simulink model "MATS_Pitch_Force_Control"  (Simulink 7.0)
settings: Solver=FixedStepDiscrete  StartTime=0.0  StopTime=inf  RelTol=1e-3
PreLoadFcn:
  | scramInitialize
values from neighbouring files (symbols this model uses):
  node = completenodestruct(node)    [scramInitialize.m]
  nTbl = 6    [scramInitialize.m]
  samplePeriod = 1/1024    (= 0.0009765625)    [scramInitialize.m]    (also in viewer.m = eval(getHeaderValue(header, 'DELTA_T')))
undefined symbols (not defined in the file or in its folder): DiscIntNeverNeededParam
libraries: xpcsystranlib x3, xpclib x2

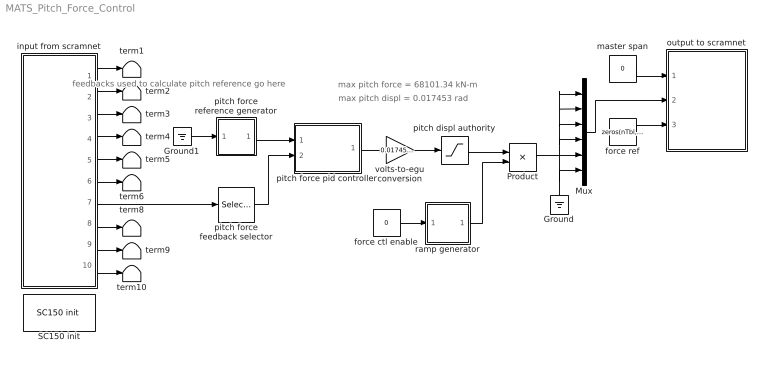
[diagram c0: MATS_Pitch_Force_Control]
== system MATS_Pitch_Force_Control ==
  note: max pitch displ = 0.017453 rad
  note: max pitch force = 68101.34 kN-m
  note: feedbacks used to calculate pitch reference go here
  Ground : Ground  Orientation=up
  Ground1 : Ground
  Mux : Mux  Inputs=nTbl
  Product : Product  OutDataType=sfix(16)  OutScaling=2^0
  SC150 init : xpcsystranlib/Shared Memory/SC150 init   node=node  pci=-1
  force ctl enable : Constant  Value=0  OutDataType=sfix(16)  OutScaling=2^0
  force ref : Constant  Value=zeros(nTbl, 1)  OutDataType=sfix(16)  OutScaling=2^0
  input from scramnet : Subsystem
  master span : Constant  Value=0  OutDataType=sfix(16)  OutScaling=2^0
  output to scramnet : Subsystem
  pitch displ authority : Saturate  UpperLimit=0.017453  LowerLimit=-0.017453  OutDataType=sfix(16)  OutScaling=2^0
  pitch force feedback selector : Selector  IndexOptions=Index vector (dialog)  Indices=5  OutputSizes=1
  pitch force pid controller : Subsystem  mask(Proportional-Integral-Derivative (PID) Controller){kp=0.1, ki=0, maxAuthority=5, kd=0, kf=0, bw=1/samplePeriod, maxUnits=68101.34, samplePeriod=samplePeriod}
      mask prompts: kp "Proportional gain"; ki "Integral gain"; maxAuthority "Max authority (percent)"; kd "Derivative gain"; kf "Feedforward gain"; bw "Bandwidth (Hz)"; maxUnits "Max units"; samplePeriod "Sample period (sec)"
  pitch force reference generator : Subsystem
  ramp generator : Subsystem  mask{rate=100}
      mask prompts: rate "Ramp rate (%/sec)"
  term{1..6,8..10} (9 alike) : Terminator
  volts-to-egu conversion : Gain  Gain=0.017453 / 10  ParameterDataType=sfix(16)  ParameterScaling=2^0  OutDataType=sfix(16)  OutScaling=2^0
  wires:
  master span/1 -> output to scramnet/1(master span)
  input from scramnet/1(master span) -> term1/1
  input from scramnet/2(displ ref) -> term2/1
  input from scramnet/3(veloc ref) -> term3/1
  input from scramnet/5(displ fbk) -> term5/1
  input from scramnet/6(veloc fbk) -> term6/1
  input from scramnet/7(force fbk) -> pitch force feedback selector/1
  input from scramnet/8(comp fbk) -> term8/1
  input from scramnet/9(press fbk) -> term9/1
  input from scramnet/10(user adcs) -> term10/1
  Ground/1 -> Mux/6, Mux/1, Mux/2, Mux/3, Mux/4
  pitch force feedback selector/1 -> pitch force pid controller/2(fbk)
  pitch force reference generator/1(out) -> pitch force pid controller/1(cmd)
  force ctl enable/1 -> ramp generator/1(inp)
  ramp generator/1(out) -> Product/2
  pitch force pid controller/1(out) -> volts-to-egu conversion/1
  volts-to-egu conversion/1 -> pitch displ authority/1
  pitch displ authority/1 -> Product/1
  Product/1 -> Mux/5
  input from scramnet/4(force ref) -> term4/1
  Ground1/1 -> pitch force reference generator/1(inp)
  Mux/1 -> output to scramnet/2(displ ref)
  force ref/1 -> output to scramnet/3(force ref)

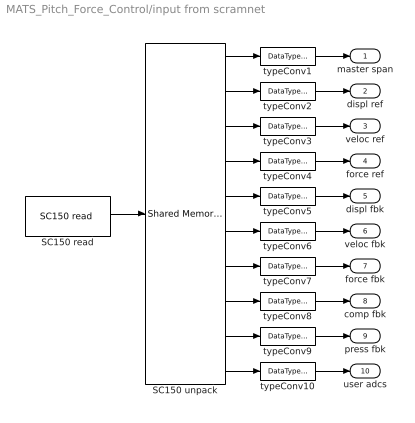
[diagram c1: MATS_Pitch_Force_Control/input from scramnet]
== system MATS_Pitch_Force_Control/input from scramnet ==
  SC150 read : xpcsystranlib/Shared Memory/SC150 read   partition=node.Partitions(4:end)  errorport=off  ts=samplePeriod  pci=-1
  SC150 unpack : xpclib/Shared Memory/Shared Memory Unpack   partition=node.Partitions(4:end)
  typeConv{1..10} (10 alike) : DataTypeConversion  OutDataTypeMode=double  OutDataType=sfix(16)  OutScaling=2^0
  master span : Outport  OutDataType=sfix(16)  OutScaling=2^0
  displ ref : Outport  Port=2  OutDataType=sfix(16)  OutScaling=2^0
  veloc ref : Outport  Port=3  OutDataType=sfix(16)  OutScaling=2^0
  force ref : Outport  Port=4  OutDataType=sfix(16)  OutScaling=2^0
  displ fbk : Outport  Port=5  OutDataType=sfix(16)  OutScaling=2^0
  veloc fbk : Outport  Port=6  OutDataType=sfix(16)  OutScaling=2^0
  force fbk : Outport  Port=7  OutDataType=sfix(16)  OutScaling=2^0
  comp fbk : Outport  Port=8  OutDataType=sfix(16)  OutScaling=2^0
  press fbk : Outport  Port=9  OutDataType=sfix(16)  OutScaling=2^0
  user adcs : Outport  Port=10  OutDataType=sfix(16)  OutScaling=2^0
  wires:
  SC150 read/1 -> SC150 unpack/1
  typeConv1/1 -> master span/1
  typeConv2/1 -> displ ref/1
  typeConv3/1 -> veloc ref/1
  typeConv4/1 -> force ref/1
  SC150 unpack/1 -> typeConv1/1
  SC150 unpack/2 -> typeConv2/1
  SC150 unpack/3 -> typeConv3/1
  SC150 unpack/4 -> typeConv4/1
  SC150 unpack/5 -> typeConv5/1
  SC150 unpack/6 -> typeConv6/1
  typeConv5/1 -> displ fbk/1
  typeConv6/1 -> veloc fbk/1
  SC150 unpack/7 -> typeConv7/1
  SC150 unpack/8 -> typeConv8/1
  SC150 unpack/9 -> typeConv9/1
  SC150 unpack/10 -> typeConv10/1
  typeConv10/1 -> user adcs/1
  typeConv9/1 -> press fbk/1
  typeConv8/1 -> comp fbk/1
  typeConv7/1 -> force fbk/1

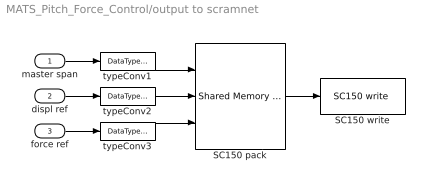
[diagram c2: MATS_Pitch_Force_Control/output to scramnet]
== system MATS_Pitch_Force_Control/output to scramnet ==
  master span : Inport  OutDataType=sfix(16)  OutScaling=2^0
  displ ref : Inport  Port=2  OutDataType=sfix(16)  OutScaling=2^0
  force ref : Inport  Port=3  OutDataType=sfix(16)  OutScaling=2^0
  SC150 pack : xpclib/Shared Memory/Shared Memory Pack   partition=node.Partitions(1:3)
  SC150 write : xpcsystranlib/Shared Memory/SC150 write   partition=node.Partitions(1:3)  errorport=off  ts=samplePeriod  pci=-1
  typeConv1 : DataTypeConversion  OutDataTypeMode=single  OutDataType=sfix(16)  OutScaling=2^0
  typeConv2 : DataTypeConversion  OutDataTypeMode=single  OutDataType=sfix(16)  OutScaling=2^0
  typeConv3 : DataTypeConversion  OutDataTypeMode=single  OutDataType=sfix(16)  OutScaling=2^0
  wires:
  master span/1 -> typeConv1/1
  displ ref/1 -> typeConv2/1
  SC150 pack/1 -> SC150 write/1
  typeConv1/1 -> SC150 pack/1
  typeConv2/1 -> SC150 pack/2
  force ref/1 -> typeConv3/1
  typeConv3/1 -> SC150 pack/3

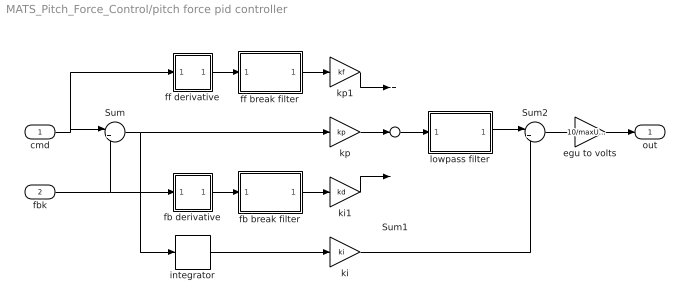
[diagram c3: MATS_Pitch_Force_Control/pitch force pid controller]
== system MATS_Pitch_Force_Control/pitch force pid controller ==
  cmd : Inport  OutDataType=sfix(16)  OutScaling=2^0
  fbk : Inport  Port=2  OutDataType=sfix(16)  OutScaling=2^0
  Sum : Sum  Inputs=|+-  OutDataType=sfix(16)  OutScaling=2^0
  Sum1 : Sum  Inputs=++-  OutDataType=sfix(16)  OutScaling=2^0
  Sum2 : Sum  Inputs=|++  OutDataType=sfix(16)  OutScaling=2^0
  egu to volts : Gain  Gain=10/maxUnits  ParameterDataType=sfix(16)  ParameterScaling=2^0  OutDataType=sfix(16)  OutScaling=2^0
  fb break filter : Subsystem  mask(First-Order Lowpass Filter){freq=bw, samplePeriod=samplePeriod}
      mask prompts: freq "Cutoff frequency (Hz)"; samplePeriod "Sample period (sec)"
      mask init:
      | bwt = freq * samplePeriod;
      | if (bwt > 0.5*0.95) 
      | 	a = [1];
      | 	b = [1];
      | else	% first-order
      | 	c	 = 1 / tan(pi * bwt);
      | 	bwt2 = 1.0 / (pi * c);	% prewarp
      | 	a    = [1 -exp(-2*pi*bwt2)];
      | 	b	 = [1] * sum(a);
      | end
  fb derivative : Subsystem  mask(Discrete Euler Derivative){samplePeriod=samplePeriod}
      mask prompts: samplePeriod "Sample period (sec)"
  ff break filter : Subsystem  mask(First-Order Lowpass Filter){freq=bw, samplePeriod=samplePeriod}
      mask prompts: freq "Cutoff frequency (Hz)"; samplePeriod "Sample period (sec)"
      mask init:
      | bwt = freq * samplePeriod;
      | if (bwt > 0.5*0.95) 
      | 	a = [1];
      | 	b = [1];
      | else	% first-order
      | 	c	 = 1 / tan(pi * bwt);
      | 	bwt2 = 1.0 / (pi * c);	% prewarp
      | 	a    = [1 -exp(-2*pi*bwt2)];
      | 	b	 = [1] * sum(a);
      | end
  ff derivative : Subsystem  mask(Discrete Euler Derivative){samplePeriod=samplePeriod}
      mask prompts: samplePeriod "Sample period (sec)"
  integrator : DiscreteIntegrator  IntegratorMethod=Integration: Backward Euler  SampleTime=-1  OutDataType=sfix(16)  OutScaling=2^0  LimitOutput=on  UpperSaturationLimit=0.01*maxAuthority*maxUnits  LowerSaturationLimit=-0.01*maxAuthority*maxUnits  ICPrevOutput=DiscIntNeverNeededParam  ICPrevScaledInput=DiscIntNeverNeededParam
  ki : Gain  Gain=ki  ParameterDataType=sfix(16)  ParameterScaling=2^0  OutDataType=sfix(16)  OutScaling=2^0
  ki1 : Gain  Gain=kd  ParameterDataType=sfix(16)  ParameterScaling=2^0  OutDataType=sfix(16)  OutScaling=2^0
  kp : Gain  Gain=kp  ParameterDataType=sfix(16)  ParameterScaling=2^0  OutDataType=sfix(16)  OutScaling=2^0
  kp1 : Gain  Gain=kf  ParameterDataType=sfix(16)  ParameterScaling=2^0  OutDataType=sfix(16)  OutScaling=2^0
  lowpass filter : Subsystem  mask(Second-order Butterworth Lowpass Filter){freq=bw, samplePeriod=samplePeriod}
      mask prompts: freq "Cutoff frequency (Hz)"; samplePeriod "Sample period (sec)"
      mask init:
      | bwt = freq * samplePeriod;
      | if (bwt > 0.5*0.95) 
      | 	a = [1];
      | 	b = [1];
      | else	% second-order butterworth 
      | 	c = 1 / tan(pi * bwt);
      | 	d = 1 + sqrt(2) * c + c^2;
      | 	a = [1 2*(1-c^2)/d (1-sqrt(2)*c+c^2)/d];
      | 	b = [1 2 1] * 0.25 * sum(a);
      | end
  out : Outport  OutDataType=sfix(16)  OutScaling=2^0
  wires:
  ki/1 -> Sum2/2
  Sum2/1 -> egu to volts/1
  ki1/1 -> Sum1/3
  fb derivative/1(out) -> fb break filter/1(inp)
  Sum/1 -> integrator/1, kp/1
  cmd/1 -> ff derivative/1(inp), Sum/1
  fbk/1 -> fb derivative/1(inp), Sum/2
  ff derivative/1(out) -> ff break filter/1(inp)
  Sum1/1 -> lowpass filter/1(inp)
  lowpass filter/1(out) -> Sum2/1
  ff break filter/1(out) -> kp1/1
  fb break filter/1(out) -> ki1/1
  kp1/1 -> Sum1/1
  kp/1 -> Sum1/2
  integrator/1 -> ki/1
  egu to volts/1 -> out/1

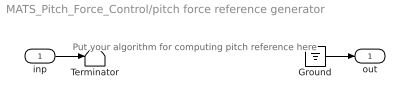
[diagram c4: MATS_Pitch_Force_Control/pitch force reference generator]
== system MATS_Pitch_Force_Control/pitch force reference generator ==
  note: Put your algorithm for computing pitch reference here
  inp : Inport  OutDataType=sfix(16)  OutScaling=2^0
  Ground : Ground
  Terminator : Terminator
  out : Outport  OutDataType=sfix(16)  OutScaling=2^0
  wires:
  inp/1 -> Terminator/1
  Ground/1 -> out/1

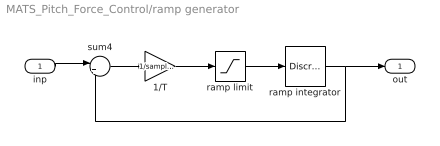
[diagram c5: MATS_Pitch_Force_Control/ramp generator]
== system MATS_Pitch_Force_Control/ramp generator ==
  inp : Inport  OutDataType=sfix(16)  OutScaling=2^0
  1/T : Gain  Gain=1/samplePeriod  ParameterDataType=sfix(16)  ParameterScaling=2^0  OutDataType=sfix(16)  OutScaling=2^0
  ramp integrator : DiscreteIntegrator  SampleTime=-1  OutDataType=sfix(16)  OutScaling=2^0  ICPrevOutput=DiscIntNeverNeededParam  ICPrevScaledInput=DiscIntNeverNeededParam
  ramp limit : Saturate  UpperLimit=rate / 100  LowerLimit=-rate / 100
  sum4 : Sum  Inputs=|+-  OutDataType=sfix(16)  OutScaling=2^0
  out : Outport  OutDataType=sfix(16)  OutScaling=2^0
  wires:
  ramp limit/1 -> ramp integrator/1
  inp/1 -> sum4/1
  1/T/1 -> ramp limit/1
  sum4/1 -> 1/T/1
  ramp integrator/1 -> sum4/2, out/1

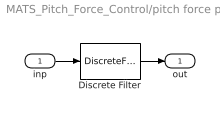
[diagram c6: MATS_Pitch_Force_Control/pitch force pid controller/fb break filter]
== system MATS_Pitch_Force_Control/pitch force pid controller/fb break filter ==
  inp : Inport  OutDataType=sfix(16)  OutScaling=2^0
  Discrete Filter : DiscreteFilter  Numerator=b  Denominator=a  SampleTime=-1
  out : Outport  OutDataType=sfix(16)  OutScaling=2^0
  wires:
  inp/1 -> Discrete Filter/1
  Discrete Filter/1 -> out/1

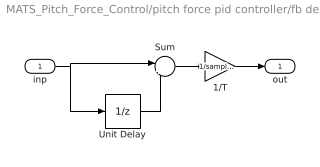
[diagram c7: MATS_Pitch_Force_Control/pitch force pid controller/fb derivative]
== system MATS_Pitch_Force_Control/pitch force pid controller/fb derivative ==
  inp : Inport  OutDataType=sfix(16)  OutScaling=2^0
  1/T : Gain  Gain=1/samplePeriod  ParameterDataType=sfix(16)  ParameterScaling=2^0  OutDataType=sfix(16)  OutScaling=2^0
  Sum : Sum  Inputs=|+-  OutDataType=sfix(16)  OutScaling=2^0
  Unit Delay : UnitDelay  SampleTime=-1
  out : Outport  OutDataType=sfix(16)  OutScaling=2^0
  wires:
  Sum/1 -> 1/T/1
  inp/1 -> Unit Delay/1, Sum/1
  Unit Delay/1 -> Sum/2
  1/T/1 -> out/1

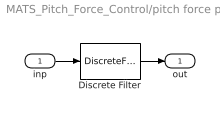
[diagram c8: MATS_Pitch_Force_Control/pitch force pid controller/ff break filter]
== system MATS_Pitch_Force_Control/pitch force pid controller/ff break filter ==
  inp : Inport  OutDataType=sfix(16)  OutScaling=2^0
  Discrete Filter : DiscreteFilter  Numerator=b  Denominator=a  SampleTime=-1
  out : Outport  OutDataType=sfix(16)  OutScaling=2^0
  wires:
  Discrete Filter/1 -> out/1
  inp/1 -> Discrete Filter/1

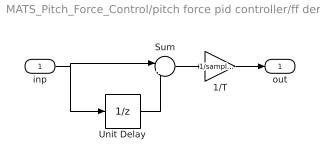
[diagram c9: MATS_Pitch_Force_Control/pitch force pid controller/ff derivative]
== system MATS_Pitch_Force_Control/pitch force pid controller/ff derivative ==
  inp : Inport  OutDataType=sfix(16)  OutScaling=2^0
  1/T : Gain  Gain=1/samplePeriod  ParameterDataType=sfix(16)  ParameterScaling=2^0  OutDataType=sfix(16)  OutScaling=2^0
  Sum : Sum  Inputs=|+-  OutDataType=sfix(16)  OutScaling=2^0
  Unit Delay : UnitDelay  SampleTime=-1
  out : Outport  OutDataType=sfix(16)  OutScaling=2^0
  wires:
  Sum/1 -> 1/T/1
  inp/1 -> Unit Delay/1, Sum/1
  Unit Delay/1 -> Sum/2
  1/T/1 -> out/1

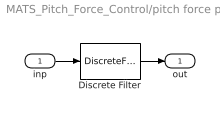
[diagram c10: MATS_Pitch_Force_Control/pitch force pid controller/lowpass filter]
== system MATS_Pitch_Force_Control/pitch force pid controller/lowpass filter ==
  inp : Inport  OutDataType=sfix(16)  OutScaling=2^0
  Discrete Filter : DiscreteFilter  Numerator=b  Denominator=a  SampleTime=-1
  out : Outport  OutDataType=sfix(16)  OutScaling=2^0
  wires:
  Discrete Filter/1 -> out/1
  inp/1 -> Discrete Filter/1
